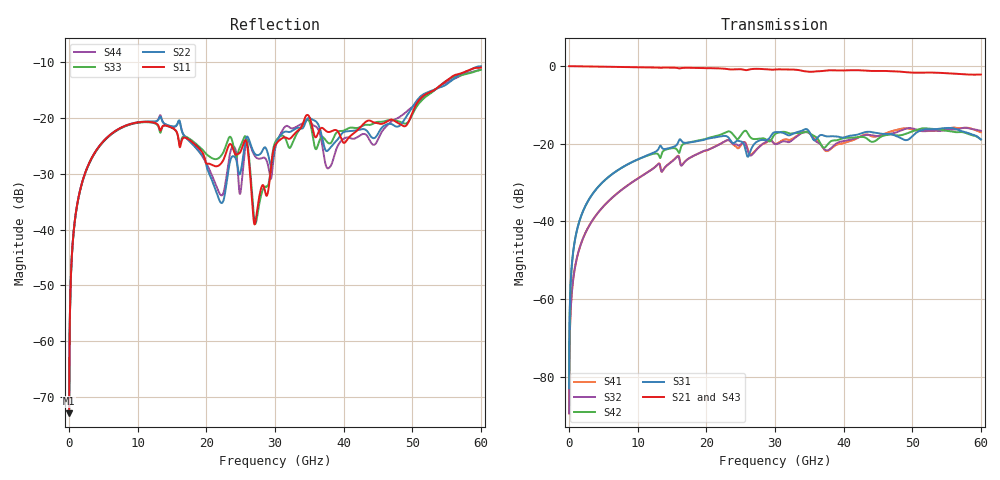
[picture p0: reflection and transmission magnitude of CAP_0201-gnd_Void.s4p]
# GHz S RI R 50
! S-Parameters data
! Freq  reS11  imS11  reS12  imS12  reS13  imS13  reS14  imS14
!  reS21  imS21  reS22  imS22  reS23  imS23  reS24  imS24
!  reS31  imS31  reS32  imS32  reS33  imS33  reS34  imS34
!  reS41  imS41  reS42  imS42  reS43  imS43  reS44  imS44
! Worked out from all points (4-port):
!   6000 points, 10 MHz to 60 GHz, reference 50 ohm
!   strongest paths, dB at 10 MHz, 15.01 GHz, 30.01 GHz, 45.01 GHz, 60 GHz:
!     S21: 0.0, -0.4, -0.9, -1.2, -2.2
!     S43: 0.0, -0.4, -0.9, -1.2, -2.1
!     S31: -82.9, -20.9, -17.0, -17.3, -18.9
!     S42: -82.9, -21.1, -17.5, -18.7, -18.9
!     S32: -89.4, -24.5, -20.1, -18.0, -16.6
!     S41: -89.4, -24.5, -20.0, -18.0, -17.0
!   lowest |S11| = -72.9 dB at 10 MHz (marker M1), VSWR 1.00, Z = 50 - j0.0106 ohm
!   |S11| at or under -10 dB: start of sweep to end of sweep
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0.01  0.0002 -0.000106  0.9998 -0.00164  1.18e-05 7.04e-05  -1.15e-05 -3.18e-05
      0.9998 -0.00164  0.0002 -0.000106  -1.15e-05 -3.18e-05  1.18e-05 7.04e-05
      1.18e-05 7.04e-05  -1.15e-05 -3.18e-05  0.0002 -0.000104  0.9998 -0.00164
      -1.15e-05 -3.18e-05  1.18e-05 7.04e-05  0.9998 -0.00164  0.0002 -0.000104
2.53  -0.0137 -0.0317  0.9232 -0.3624  0.00603 0.0157  -0.00234 -0.00719
      0.9232 -0.3624  -0.0137 -0.0317  -0.00234 -0.00719  0.00606 0.0157
      0.00603 0.0157  -0.00234 -0.00719  -0.0135 -0.0314  0.9231 -0.3625
      -0.00234 -0.00719  0.00606 0.0157  0.9231 -0.3625  -0.0136 -0.0314
13.24  -0.0723 0.0298  -0.3266 -0.8923  0.0901 -0.0255  -0.0468 0.0263
       -0.3266 -0.8923  -0.0973 0.033  -0.0464 0.0261  0.0623 -0.0219
       0.0901 -0.0255  -0.0464 0.0261  -0.07 0.0269  -0.3257 -0.8885
       -0.0468 0.0263  0.0623 -0.0219  -0.3257 -0.8885  -0.1001 0.0336
27.08  -0.00791 0.00797  -0.6796 0.6253  -0.0612 -0.081  0.0665 0.0461
       -0.6796 0.6253  -0.0417 0.0233  0.0654 0.0455  -0.0957 -0.0638
       -0.0612 -0.081  0.0654 0.0455  -0.00478 0.0104  -0.6843 0.6203
       0.0665 0.0461  -0.0957 -0.0638  -0.6843 0.6203  -0.037 0.0266
32.27  -0.0611 0.0247  -0.0537 0.9036  -0.13 0.00174  0.1099 -0.0259
       -0.0537 0.9036  -0.0604 0.0452  0.1054 -0.021  -0.1337 0.0221
       -0.13 0.00174  0.1054 -0.021  -0.0474 0.0275  -0.0677 0.8943
       0.1099 -0.0259  -0.1337 0.0221  -0.0677 0.8943  -0.06 0.0549
45.05  0.0562 0.0698  0.8508 -0.1794  0.0617 0.1219  -0.0607 -0.1104
       0.8508 -0.1794  0.0387 0.062  -0.0679 -0.1061  0.0281 0.1129
       0.0617 0.1219  -0.0679 -0.1061  0.0616 0.069  0.8524 -0.1636
       -0.0607 -0.1104  0.0281 0.1129  0.8524 -0.1636  0.0274 0.0591
60  0.1509 -0.24  -0.58 -0.5225  0.0255 -0.1112  -0.0141 0.1403
    -0.58 -0.5225  0.1622 -0.2424  -0.0179 0.1461  0.0298 -0.1097
    0.0255 -0.1112  -0.0179 0.1461  0.1464 -0.2274  -0.5823 -0.5251
    -0.0141 0.1403  0.0298 -0.1097  -0.5823 -0.5251  0.1495 -0.2266
